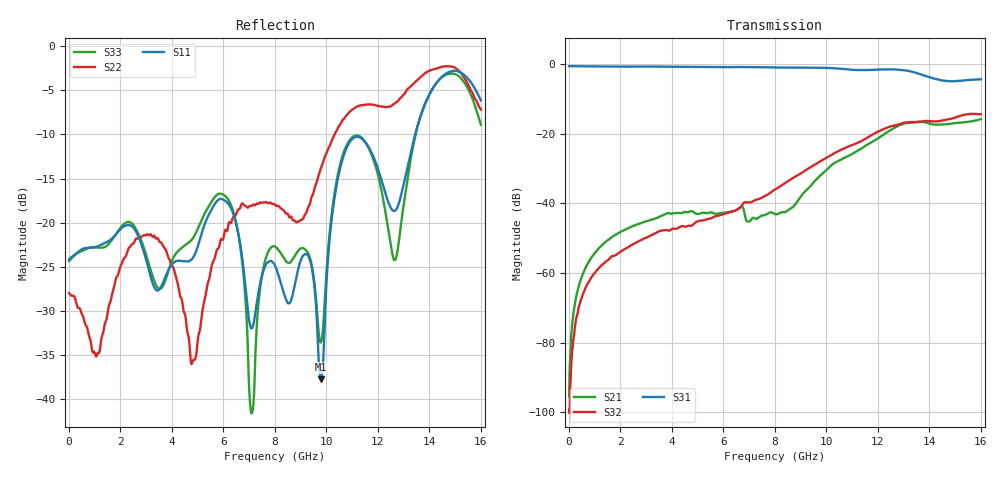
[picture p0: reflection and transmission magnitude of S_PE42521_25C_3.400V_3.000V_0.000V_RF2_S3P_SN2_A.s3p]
! Device ID: PE42521_Char_Units
! Serial: 2
! Insertion: A
! Temp: 25C
! VDD: 3.400
! Control_Hi: 3.000
! Control_Lo: 0.000
! Logic State: RF2
! ThroughPath: 3-1
! Port 1: RFC
! Port 2: RF1
! Port 3: RF2
! V1 = 3.00
! V2 = 3.00
! V3 = 0.00
! IDD: 1.359909e-04
! FILE NAME
! DATE 07-24-2013 19:16:06
! CORRECTED  DATA
#  Hz  S  RI  R  50
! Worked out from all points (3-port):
!   801 points, 10 MHz to 16.01 GHz, reference 50 ohm
!   strongest paths, dB at 10 MHz, 4.01 GHz, 8.01 GHz, 12.01 GHz, 16.01 GHz:
!     S31: -0.6, -0.8, -1.0, -1.6, -4.4
!     S32: -99.2, -47.3, -36.0, -19.4, -14.4
!     S21: -95.5, -42.9, -43.1, -21.4, -15.8
!   lowest |S11| = -37.7 dB at 9.79 GHz (marker M1), VSWR 1.03, Z = 51.2 + j0.547 ohm
!   |S11| at or under -10 dB: start of sweep to 13.46 GHz
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1e7  0.0618 -0.000139  -5.32e-06 -4.89e-06  0.9299 -0.00288
     1.27e-05 -1.11e-05  -0.0399 0.000206  -4.92e-06 -7.08e-06
     0.9305 -0.00292  2.69e-06 -1.07e-05  0.0606 -0.000555
1.75e9  0.0803 0.0226  0.000721 0.00336  0.8344 -0.382
        0.000726 0.00337  0.00283 0.0429  7.33e-05 0.00176
        0.8354 -0.3814  6.74e-05 0.00176  0.0805 0.0191
4.83e9  0.041 -0.0486  0.00558 0.00507  0.3447 -0.8397
        0.00556 0.00511  -0.000468 -0.0166  0.00083 0.00492
        0.3466 -0.8401  0.000817 0.0049  0.0433 -0.0696
6.15e9  0.129 -0.0164  0.00511 0.00535  0.0626 -0.8988
        0.00509 0.00537  0.0619 0.0648  0.00122 0.0072
        0.0652 -0.8986  0.00121 0.00717  0.1323 -0.039
7.11e9  -0.00298 -0.025  0.00374 0.00468  -0.162 -0.8898
        0.00374 0.0047  -0.00175 0.1248  0.00146 0.0104
        -0.1587 -0.89  0.00141 0.0104  -0.00248 -0.00795
8.01e9  -0.0565 -0.00859  0.00294 0.00642  -0.3572 -0.8168
        0.00293 0.00638  -0.0778 0.0996  0.0015 0.0157
        -0.3546 -0.8188  0.00146 0.0158  -0.0733 0.000124
9.79e9  0.0119 0.00534  -0.00344 0.0252  -0.686 -0.5528
        -0.00349 0.0252  0.00677 0.2032  0.0176 0.0365
        -0.6858 -0.5557  0.0175 0.0366  0.0205 0.00422
1.087e10  -0.1027 0.2599  0.014 0.046  -0.7786 -0.2988
          0.0139 0.046  -0.0145 0.4178  0.0504 0.0422
          -0.7786 -0.3016  0.0502 0.0425  -0.0501 0.2832
1.267e10  0.0601 0.1002  0.1077 0.0576  -0.823 0.1255
          0.1076 0.058  0.3282 0.3428  0.1295 -0.0249
          -0.8256 0.122  0.1298 -0.0241  0.0274 0.0549
1.601e10  0.4258 0.2476  0.0548 -0.1527  -0.3755 0.4715
          0.056 -0.1523  0.3956 0.186  -0.0621 -0.1811
          -0.3778 0.4714  -0.0597 -0.1812  0.2972 0.2015
